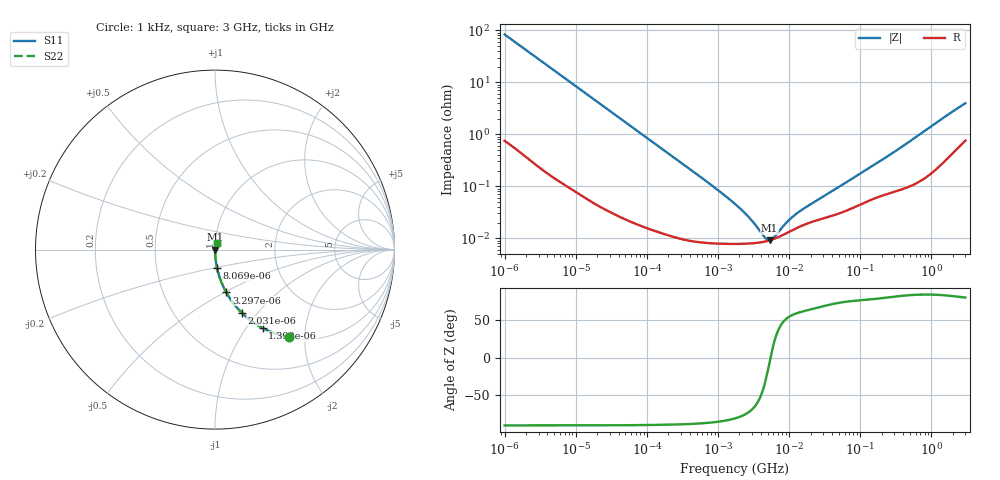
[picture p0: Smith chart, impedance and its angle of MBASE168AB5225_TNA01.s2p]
! MBASE168AB5225_TNA01  S-PARAMETER MODEL  ( Standard Model )
! Model Generated by TAIYO YUDEN Corporation (http://www.ty-top.com)
! Version 1.0
! TAIYO YUDEN Control No. 220601
! Copyright(c) 2012 TAIYO YUDEN CO.,LTD. All Rights Reserved.
! Product Description (link to TY-COMPAS)
! https://ds.yuden.co.jp/TYCOMPAS/or/detail?pn=MBASE168AB5225KTNA01&u=M
! Products Name : Multilayer Ceramic Capacitors
! Characteristics :
!  Capacitance : 2.2 [uF] , Rated Voltage : 16 [V] , TCC : X5R
!  Case Size : 1.6 x 0.8 / 0.063 x 0.031 [mm/inch] , Thickness : 0.8 / 0.031 [mm/inch]
!  (Conditions: Temperature = 25 [degC] , DC Bias Voltage = 0 [V])
! External Node Assignments :
!  1  o---| |---o  2
! GND o---------o GND
! Frequency Range : 1kHz  -  3GHz  [ 401 STEP ]
# MHZ S RI R 50
! Freq[MHz].  S11 Real  S11 Imag  S21 Real  S21 Imag  S12 Real  S12 Imag  S22 Real  S22 Imag
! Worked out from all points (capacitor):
!   401 points, 1 kHz to 3 GHz, reference 50 ohm
!   read as one part in series: C = 1.9 uF near 1.077 kHz
!   lowest |Z| = 9.16 mohm at 5.301 MHz (marker M1)
!   series resonance near 5.474 MHz, so ESL is about 440 pH
!   S11 on the Smith chart (normalised r, x): 1 kHz: 1.01, -1.67; 1.399 kHz: 1.01, -1.20; 2.031 kHz: 1.01, -0.83; 3.297 kHz: 1.00, -0.51; 8.069 kHz: 1.00, -0.21; 3 GHz: 1.02, +0.08
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0.001  0.4116 -0.4877  0.5884 0.4877  0.5884 0.4877  0.4116 -0.4877
0.001399  0.2656 -0.4372  0.7344 0.4372  0.7344 0.4372  0.2656 -0.4372
0.002031  0.148 -0.3507  0.852 0.3507  0.852 0.3507  0.148 -0.3507
0.003297  0.0628 -0.2385  0.9372 0.2385  0.9372 0.2385  0.0628 -0.2385
0.008069  0.0117 -0.1034  0.9883 0.1034  0.9883 0.1034  0.0117 -0.1034
0.01216  0.00547 -0.0692  0.9945 0.0692  0.9945 0.0692  0.00547 -0.0692
0.033275  0.000952 -0.0255  0.999 0.0255  0.999 0.0255  0.000952 -0.0255
0.147855  0.000164 -0.00581  0.9998 0.00581  0.9998 0.00581  0.000164 -0.00581
0.762639  8.16e-05 -0.00111  0.9999 0.00111  0.9999 0.00111  8.16e-05 -0.00111
1.732051  7.79e-05 -0.000451  0.9999 0.000451  0.9999 0.000451  7.79e-05 -0.000451
2.812335  7.92e-05 -0.000227  0.9999 0.000227  0.9999 0.000227  7.92e-05 -0.000227
4.399271  8.54e-05 -6.93e-05  0.9999 6.93e-05  0.9999 6.93e-05  8.54e-05 -6.93e-05
4.739869  8.74e-05 -4.53e-05  0.9999 4.53e-05  0.9999 4.53e-05  8.74e-05 -4.53e-05
5.30084  9.11e-05 -9.97e-06  0.9999 9.97e-06  0.9999 9.97e-06  9.11e-05 -9.97e-06
5.928204  9.58e-05 2.47e-05  0.9999 -2.47e-05  0.9999 -2.47e-05  9.58e-05 2.47e-05
6.387174  9.95e-05 4.75e-05  0.9999 -4.75e-05  0.9999 -4.75e-05  9.95e-05 4.75e-05
8.933959  0.000123 0.000148  0.9999 -0.000148  0.9999 -0.000148  0.000123 0.000148
11.59828  0.000147 0.000226  0.9999 -0.000226  0.9999 -0.000226  0.000147 0.000226
21.06097  0.000207 0.000423  0.9998 -0.000423  0.9998 -0.000423  0.000207 0.000423
256.0921  0.000747 0.0039  0.9993 -0.0039  0.9993 -0.0039  0.000747 0.0039
1780.008  0.0043 0.0244  0.9957 -0.0244  0.9957 -0.0244  0.0043 0.0244
3000  0.009 0.0383  0.991 -0.0383  0.991 -0.0383  0.009 0.0383
